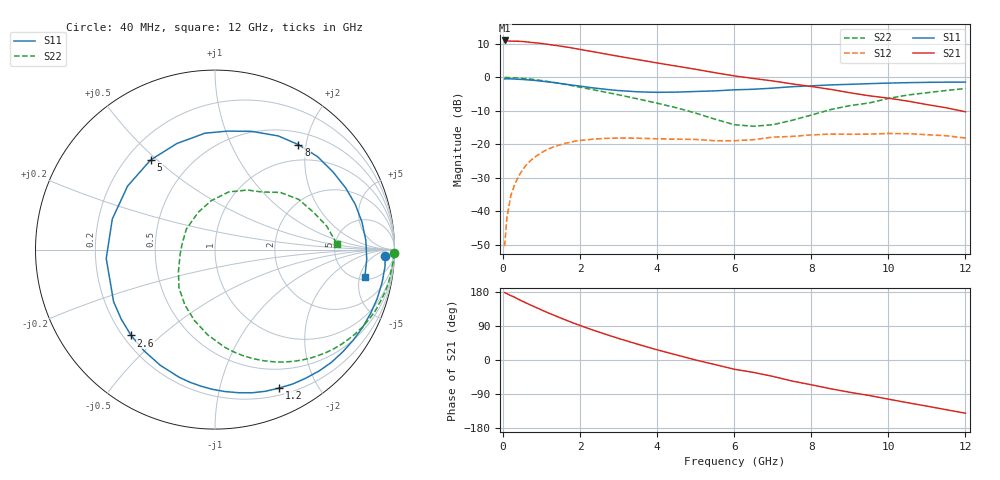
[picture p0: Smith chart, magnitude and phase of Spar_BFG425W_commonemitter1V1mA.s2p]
! Filename: 11bfg425.001
! BFG425W Field C1
! V1=7.910E-001V,V2=1.000E+000V, I1=1.367E-005A, I2=1.000E-003A
# GHz  S  MA  R 50
!  S11  S21  S12  S22
!Freq(GHz)  Mag  Ang  Mag  Ang  Mag  Ang  Mag  Ang
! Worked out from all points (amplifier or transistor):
!   44 points, 40 MHz to 12 GHz, reference 50 ohm
!   highest |S21| = 11.0 dB at 40 MHz (marker M1)
!   |S21| within 3 dB of that: start of sweep to 2.157 GHz
!   unconditionally stable (mu >= 1): 3.416 GHz to end of sweep
!   at 700 MHz: K = 0.13, MSG = 17.8 dB, |S12| = -25.0 dB
!   at 2.4 GHz: K = 0.58, MSG = 13.0 dB, |S12| = -18.4 dB
!   at 12 GHz: K = 2.18, MAG = -2.2 dB, |S12| = -18.1 dB
!   S11 on the Smith chart (normalised r, x): 40 MHz: 26, -17; 1.2 GHz: 0.27, -1.53; 2.6 GHz: 0.23, -0.40; 5 GHz: 0.30, +0.48; 8 GHz: 0.70, +1.86; 12 GHz: 5.45, -6.04
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0.04  0.948 -2.0  3.56 177.8  0.003 83.3  0.996 -1.2
0.1  0.952 -5.5  3.502 175.1  0.008 87.1  0.996 -3.4
0.2  0.949 -11.1  3.478 169.9  0.017 81.9  0.988 -7.2
0.3  0.944 -16.7  3.471 165.7  0.025 77.9  0.985 -10.6
0.5  0.93 -27.6  3.44 155.3  0.041 69.9  0.965 -17.5
0.7  0.912 -38.6  3.339 145.7  0.056 62.0  0.942 -24.4
1  0.877 -54.7  3.206 132.0  0.075 51.0  0.895 -34.0
1.2  0.85 -65.2  3.092 123.2  0.086 44.1  0.861 -40.0
1.7  0.779 -90.9  2.808 102.6  0.106 28.4  0.768 -53.9
2.2  0.713 -115.3  2.495 83.7  0.117 15.0  0.677 -66.2
2.6  0.669 -134.3  2.269 69.9  0.122 5.9  0.61 -75.4
3  0.635 -152.9  2.063 56.8  0.124 -2.0  0.548 -84.2
3.5  0.608 -175.4  1.84 41.5  0.123 -10.3  0.476 -95.0
4  0.597 163.4  1.642 26.9  0.121 -17.3  0.411 -106.2
4.5  0.602 144.0  1.472 13.4  0.119 -22.7  0.351 -118.6
5  0.615 125.7  1.319 0.0  0.118 -28.5  0.292 -133.5
6  0.651 94.9  1.052 -24.3  0.113 -37.1  0.196 -172.4
6.5  0.664 83.9  0.962 -32.8  0.117 -32.1  0.186 170.5
8  0.747 51.5  0.73 -65.4  0.138 -50.6  0.273 94.5
8.5  0.771 42.2  0.662 -75.8  0.142 -58.3  0.33 76.7
10.5  0.833 10.7  0.442 -112.7  0.144 -89.0  0.544 30.9
12  0.849 -10.5  0.306 -140.4  0.124 -118.7  0.681 2.4
